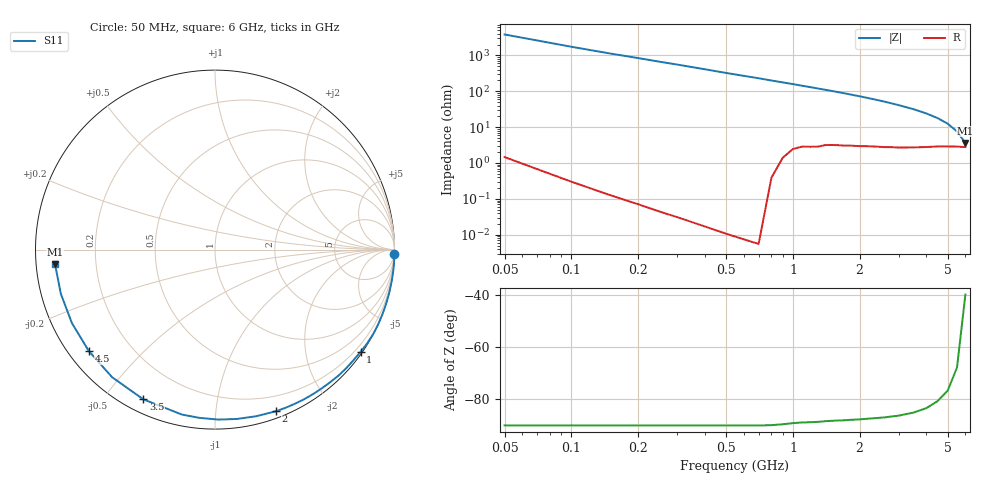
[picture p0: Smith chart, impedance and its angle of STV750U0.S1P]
! SIEMENS Discrete & RF Semiconductors
! BA892
! Si PIN Diode in SCD-80
! VR = 0.75 V
! S-Parameters:  September  1997
# GHz  S  MA  R  50
!  f  S11
! GHz  MAG  ANG
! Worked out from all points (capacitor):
!   34 points, 50 MHz to 6 GHz, reference 50 ohm
!   read as one part to ground: C = 917 fF near 50 MHz
!   lowest |Z| = 3.61 ohm at 6 GHz (marker M1)
!   S11 on the Smith chart (normalised r, x): 50 MHz: 0, -76; 1 GHz: 0.05, -3.16; 2 GHz: 0.06, -1.45; 3.5 GHz: 0.05, -0.63; 4.5 GHz: 0.06, -0.35; 6 GHz: 0.06, -0.05
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0.05  1 -1.5
0.2  1 -6.8
0.3  1 -10.3
0.4  1 -13.9
0.5  1 -17.6
0.6  1 -21.1
0.7  1 -24.5
0.8  0.9991 -28.2
0.9  0.9958 -31.7
1  0.9911 -35.1
1.1  0.9875 -38.7
1.2  0.9855 -42.1
1.3  0.9829 -45.6
1.5  0.9756 -52.3
1.6  0.9729 -55.8
1.8  0.9674 -62.6
2  0.9625 -69.3
2.2  0.9565 -76.0
2.4  0.9515 -82.6
2.6  0.9471 -88.9
2.8  0.9415 -95.2
3  0.9375 -101.3
3.5  0.925 -115.6
4  0.9132 -128.9
4.5  0.902 -141.2
5  0.8962 -152.8
5.5  0.8935 -164.0
6  0.8949 -174.7
